|Texas Instruments Incorporated
| IBIS Model of : TMUX6213
| 48V 4x1:1 Analog Switch Array
| This file contains package information for the following:
|  TSSOP 16-pin (PW) package as [Component] TMUX6213_PW
|  QFN 16-pin (RUM) package as [Component] TMUX6213_RUM
| This device can be powered at the following Vccs:
| Single Rail Supply Configurations:
|  5.0 volt VDD, 0V VSS
|  12.0 volt VDD, 0V VSS
|  36.0 volt VDD, 0V VSS
| Dual Rail Supply Configurations:
|  5.0 volt VDD, -5V VSS
|  15.0 volt VDD, -15V VSS
| Digital Voltage Range : 4.5-38.5
[IBIS Ver] 4.1
[File name] tmux6213.ibs
[File Rev] 1.0
[Date] 12/30/2020
[Source]
| Texas Instruments Incorporated.
| 12500 TI Blvd
| Dallas, TX -75243
[Notes] Revision History:
| Rev 1.0: 12/30/2020
| - Initial version of the model
| - Model generated from simulations in TISPICE/SPECTRE
| - C_comp although listed in numerical order of value are
| obtained from varying PVT conditions. For PVT conditions for
| each specific value refer the buffer description under
| respective [Model]. IBIS model user is responsible for using
| appropriate C_comp to simulate for Signal Integrity.
| - Warnings regarding combined Non-monotonicity of various models have been
| reviewed and considered minor and can be ignored.
|**** Modify the following if you use [Model Selector]***********
| - Model names with a trailing voltage extension contain the model for
| operation at that voltage range.
[Disclaimer]
| This model is designed as an aid for customers of Texas Instruments.
| TI and its licensors and suppliers make no warranties, either expressed
| or implied, with respect to this model, including the warranties of
| merchantability or fitness for a particular purpose. The model is
| provided solely on an "as is" basis. The entire risk as to its quality
| and performance is with the customer.
| This model is subject to change without notice. Texas Instruments
| Incorporated is not responsible for updating this model.
[Copyright]
(C) Copyright 2020 Texas Instruments Incorporated. All rights reserved.
| Component TMUX6213_DGK 8-pin SOT (per package)
[Component] TMUX6213_PW
[Manufacturer]  Texas Instruments Incorporated
[Package] |TSSOP (PW) 16-pin
| variable typ min max
R_pkg 0.05 0.04 0.06
L_pkg 1.0nH 0.8nH 1.2nH
C_pkg 0.2pF 0.16pF 0.24pF
| pin number (pin name) mapping to model name
[Pin] signal_name   model_name   R_pin L_pin C_pin
1   IN1 		INPUT_PD   NA   NA   NA
2   D1   TMUX6213_DX   NA   NA   NA
3   S1   TMUX6213_SX   NA   NA   NA
4   VSS   POWER   NA   NA   NA
5   GND 		GND   NA   NA   NA
6   S4   TMUX6213_SX   NA   NA   NA
7   D4   TMUX6213_DX   NA   NA   NA
8   IN4 		INPUT_PD   NA   NA   NA
9   IN3 		INPUT_PD   NA   NA   NA
10   D3   TMUX6213_DX   NA   NA   NA
11   S3   TMUX6213_SX   NA   NA   NA
12   NC   NC   NA   NA   NA
13   VDD 		POWER   NA   NA   NA
14   S2   TMUX6213_SX   NA   NA   NA
15   D2   TMUX6213_DX   NA   NA   NA
16   IN2 		INPUT_PD   NA   NA   NA
[Series Switch Groups]
| Function Group States
On  1 /   | S1->D1 IN HIGH
Off  /   | EN LOW
[Series Pin Mapping]   pin_2   model_name   function_table_group
| PW Package
|2   3   TMUX6213_SX_SINGLE_5V_S   1
|3   2   TMUX6213_DX_SINGLE_5V_S   1
|15   14   TMUX6213_SX_SINGLE_5V_S   1
|14   15   TMUX6213_DX_SINGLE_5V_S   1
|7   6   TMUX6213_SX_SINGLE_5V_S   1
|6   7   TMUX6213_DX_SINGLE_5V_S   1
|10   11   TMUX6213_SX_SINGLE_5V_S   1
|11   10   TMUX6213_DX_SINGLE_5V_S   1
|2   3   TMUX6213_SX_SINGLE_12V_S   1
|3   2   TMUX6213_DX_SINGLE_12V_S   1
|15   14   TMUX6213_SX_SINGLE_12V_S   1
|14   15   TMUX6213_DX_SINGLE_12V_S   1
|7   6   TMUX6213_SX_SINGLE_12V_S   1
|6   7   TMUX6213_DX_SINGLE_12V_S   1
|10   11   TMUX6213_SX_SINGLE_12V_S   1
|11   10   TMUX6213_DX_SINGLE_12V_S   1
|2   3   TMUX6213_SX_SINGLE_36V_S   1
|3   2   TMUX6213_DX_SINGLE_36V_S   1
|15   14   TMUX6213_SX_SINGLE_36V_S   1
|14   15   TMUX6213_DX_SINGLE_36V_S   1
|7   6   TMUX6213_SX_SINGLE_36V_S   1
|6   7   TMUX6213_DX_SINGLE_36V_S   1
|10   11   TMUX6213_SX_SINGLE_36V_S   1
|11   10   TMUX6213_DX_SINGLE_36V_S   1
2   3   TMUX6213_SX_DUAL_PM5_S   1
3   2   TMUX6213_DX_DUAL_PM5_S   1
15   14   TMUX6213_SX_DUAL_PM5_S   1
14   15   TMUX6213_DX_DUAL_PM5_S   1
7   6   TMUX6213_SX_DUAL_PM5_S   1
6   7   TMUX6213_DX_DUAL_PM5_S   1
10   11   TMUX6213_SX_DUAL_PM5_S   1
11   10   TMUX6213_DX_DUAL_PM5_S   1
|2   3   TMUX6213_SX_DUAL_PM15_S   1
|3   2   TMUX6213_DX_DUAL_PM15_S   1
|15   14   TMUX6213_SX_DUAL_PM15_S   1
|14   15   TMUX6213_DX_DUAL_PM15_S   1
|7   6   TMUX6213_SX_DUAL_PM15_S   1
|6   7   TMUX6213_DX_DUAL_PM15_S   1
|10   11   TMUX6213_SX_DUAL_PM15_S   1
|11   10   TMUX6213_DX_DUAL_PM15_S   1
| Component TMUX6213_RUM 16-pin QFN (per package)
[Component] TMUX6213_RUM
[Manufacturer]  Texas Instruments Incorporated
[Package] |QFN (RUM) 16-pin
| variable typ 		min 		max
R_pkg 	0.05 		0.04 		0.06
L_pkg 	1.0nH 	0.8nH 	1.2nH
C_pkg 	0.2pF 	0.16pF 	0.24pF
| pin number (pin name) mapping to model name
[Pin] signal_name   model_name   R_pin L_pin C_pin
1   S1   TMUX6213_SX   NA   NA   NA
2   VSS   POWER   NA   NA   NA
3   GND 		GND   NA   NA   NA
4   S4   TMUX6213_SX   NA   NA   NA
5   D4   TMUX6213_DX   NA   NA   NA
6   IN4 		INPUT_PD   NA   NA   NA
7   IN3 		INPUT_PD   NA   NA   NA
8   D3   TMUX6213_DX   NA   NA   NA
9   S3   TMUX6213_SX   NA   NA   NA
10   NC   NC   NA   NA   NA
11   VDD 		POWER   NA   NA   NA
12   S2   TMUX6213_SX   NA   NA   NA
13   D2   TMUX6213_DX   NA   NA   NA
14   IN2 		INPUT_PD   NA   NA   NA
15   IN1 		INPUT_PD   NA   NA   NA
16   D1   TMUX6213_DX   NA   NA   NA
[Series Switch Groups]
| Function Group States
|On  1 /   | S1->D1 IN HIGH
|Off  /   | EN LOW
[Series Pin Mapping]   pin_2   model_name   function_table_group
| RUM Package
|16   1   TMUX6213_SX_SINGLE_5V_S   1
|1   16   TMUX6213_DX_SINGLE_5V_S   1
|13   12   TMUX6213_SX_SINGLE_5V_S   1
|12   13   TMUX6213_DX_SINGLE_5V_S   1
|8   8   TMUX6213_SX_SINGLE_5V_S   1
|9   9   TMUX6213_DX_SINGLE_5V_S   1
|5   4   TMUX6213_SX_SINGLE_5V_S   1
|4   5   TMUX6213_DX_SINGLE_5V_S   1
|16   1   TMUX6213_SX_SINGLE_12V_S   1
|1   16   TMUX6213_DX_SINGLE_12V_S   1
|13   12   TMUX6213_SX_SINGLE_12V_S   1
|12   13   TMUX6213_DX_SINGLE_12V_S   1
|8   8   TMUX6213_SX_SINGLE_12V_S   1
|9   9   TMUX6213_DX_SINGLE_12V_S   1
|5   4   TMUX6213_SX_SINGLE_12V_S   1
|4   5   TMUX6213_DX_SINGLE_12V_S   1
|16   1   TMUX6213_SX_SINGLE_36V_S   1
|1   16   TMUX6213_DX_SINGLE_36V_S   1
|13   12   TMUX6213_SX_SINGLE_36V_S   1
|12   13   TMUX6213_DX_SINGLE_36V_S   1
|8   8   TMUX6213_SX_SINGLE_36V_S   1
|9   9   TMUX6213_DX_SINGLE_36V_S   1
|5   4   TMUX6213_SX_SINGLE_36V_S   1
|4   5   TMUX6213_DX_SINGLE_36V_S   1
|16   1   TMUX6213_SX_DUAL_PM5_S   1
|1   16   TMUX6213_DX_DUAL_PM5_S   1
|13   12   TMUX6213_SX_DUAL_PM5_S   1
|12   13   TMUX6213_DX_DUAL_PM5_S   1
|8   8   TMUX6213_SX_DUAL_PM5_S   1
|9   9   TMUX6213_DX_DUAL_PM5_S   1
|5   4   TMUX6213_SX_DUAL_PM5_S   1
|4   5   TMUX6213_DX_DUAL_PM5_S   1
|16   1   TMUX6213_SX_DUAL_PM15_S   1
|1   16   TMUX6213_DX_DUAL_PM15_S   1
|13   12   TMUX6213_SX_DUAL_PM15_S   1
|12   13   TMUX6213_DX_DUAL_PM15_S   1
|8   8   TMUX6213_SX_DUAL_PM15_S   1
|9   9   TMUX6213_DX_DUAL_PM15_S   1
|5   4   TMUX6213_SX_DUAL_PM15_S   1
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[Model Selector] INPUT_PU
INBUF_PU_5V   INPUT_PU   buffer at 5V operation.
INBUF_PU_12V   INPUT_PU   buffer at 12V operation.
INBUF_PU_15V   INPUT_PU   buffer at 15V operation.
INBUF_PU_20V   INPUT_PU   buffer at 20V operation.
INBUF_PU_36V   INPUT_PU   buffer at 36V operation.
[Model Selector] INPUT_PD
INBUF_PD_5V   INPUT_PD   buffer at 5V operation.
INBUF_PD_12V   INPUT_PD   buffer at 12V operation.
INBUF_PD_15V   INPUT_PD   buffer at 15V operation.
INBUF_PD_20V   INPUT_PD   buffer at 20V operation.
INBUF_PD_36V   INPUT_PD   buffer at 36V operation.
[Model Selector] TMUX6213_SX
TMUX6213_SX_SINGLE_5V  switch termination at +5V operation.
TMUX6213_SX_SINGLE_12V  switch termination at +12V operation.
TMUX6213_SX_SINGLE_36V  switch termination at +36V operation.
TMUX6213_SX_DUAL_PM5  switch termination at +/-5V operation.
TMUX6213_SX_DUAL_PM15  switch termination at +/-15V operation.
[Model Selector] TMUX6213_SX_S
TMUX6213_SX_SINGLE_5V_S  switch at +5V operation.
TMUX6213_SX_SINGLE_12V_S  switch at +12V operation.
TMUX6213_SX_SINGLE_36V_S  switch at +36V operation.
TMUX6213_SX_DUAL_PM5_S  switch at +/-5V operation.
TMUX6213_SX_DUAL_PM15_S  switch at +/-15V operation.
[Model Selector] TMUX6213_DX
TMUX6213_DX_SINGLE_5V  termination switch at +5V operation.
TMUX6213_DX_SINGLE_12V  termination switch at +12V operation.
TMUX6213_DX_SINGLE_36V  termination switch at +36V operation.
TMUX6213_DX_DUAL_PM5	termination switch at +/-15V operation.
TMUX6213_DX_DUAL_PM15  termination switch at +/-15V operation.
[Model Selector] TMUX6213_DX_S
TMUX6213_DX_SINGLE_5V_S  switch at +5V operation.
TMUX6213_DX_SINGLE_12V_S  switch at +12V operation.
TMUX6213_DX_SINGLE_36V_S  switch at +36V operation.
TMUX6213_DX_DUAL_PM5_S  switch at +/-5V operation.
TMUX6213_DX_DUAL_PM15_S  switch at +/-15V operation.
| Model12
[Model]   TMUX6213_SX_SINGLE_5V_S
Model_type  Series_switch
| variable   typ   min   max
C_comp   0   0   0
[Temperature Range]   25   125   -40
| Ambient temperature   25   125   -40
[Voltage range]   5   4.5   5.5
[On]
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[Off]
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[Model]   TMUX6213_DX_SINGLE_5V_S
Model_type  Series_switch
| variable   typ   min   max
C_comp   0   0   0
[Temperature Range]   25   125   -40
| Ambient temperature   25   125   -40
[Voltage range]   5   5   5
[On]
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[Off]
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[Model]   TMUX6213_SX_SINGLE_12V_S
Model_type  Series_switch
| variable   typ   min   max
C_comp   0   0   0
[Temperature Range]   25   125   -40
| Ambient temperature   25   125   -40
[Voltage range]   12   12   12
[On]
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[Off]
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[Model]   TMUX6213_DX_SINGLE_12V_S
Model_type  Series_switch
| variable   typ   min   max
C_comp   0   0   0
[Temperature Range]   25   125   -40
| Ambient temperature   25   125   -40
[Voltage range]   12   12   12
[On]
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[Off]
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[Model]   TMUX6213_SX_SINGLE_36V_S
Model_type  Series_switch
| variable   typ   min   max
C_comp   0   0   0
[Temperature Range]   25   125   -40
| Ambient temperature   25   125   -40
[Voltage range]   36   36   36
[On]
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[Off]
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[Model]   TMUX6213_DX_SINGLE_36V_S
Model_type  Series_switch
| variable   typ   min   max
C_comp   0   0   0
[Temperature Range]   25   125   -40
| Ambient temperature   25   125   -40
[Voltage range]   36   36   36
[On]
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[Off]
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[Model]   TMUX6213_SX_DUAL_PM5_S
Model_type  Series_switch
| variable   typ   min   max
C_comp   0   0   0
[Temperature Range]   25   125   -40
| Ambient temperature   25   125   -40
[Voltage range]   0   -5   5
[On]
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[Off]
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[Model]   TMUX6213_DX_DUAL_PM5_S
Model_type  Series_switch
| variable   typ   min   max
C_comp   0   0   0
[Temperature Range]   25   125   -40
| Ambient temperature   25   125   -40
[Voltage range]   0   -5   5
[On]
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[Off]
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[Model]   TMUX6213_SX_DUAL_PM15_S
Model_type  Series_switch
| variable   typ   min   max
C_comp   0   0   0
[Temperature Range]   25   125   -40
| Ambient temperature   25   125   -40
[Voltage range]   0   -15   15
[On]
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[Off]
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[Model]   TMUX6213_DX_DUAL_PM15_S
Model_type  Series_switch
| variable   typ   min   max
C_comp   0   0   0
[Temperature Range]   25   125   -40
| Ambient temperature   25   125   -40
[Voltage range]   0   -15   15
[On]
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[Off]
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| Models and submodels in the file (30): INBUF_PD_5V (Input), INBUF_PD_12V (Input), INBUF_PD_15V (Input), INBUF_PD_20V (Input), INBUF_PD_36V (Input), INBUF_PU_5V (Input), INBUF_PU_12V (Input), INBUF_PU_15V (Input), INBUF_PU_20V (Input), INBUF_PU_36V (Input), TMUX6213_SX_SINGLE_5V_S (Series_switch), TMUX6213_SX_SINGLE_5V (Terminator), TMUX6213_DX_SINGLE_5V_S (Series_switch), TMUX6213_DX_SINGLE_5V (Terminator), TMUX6213_SX_SINGLE_12V_S (Series_switch), TMUX6213_SX_SINGLE_12V (Terminator), TMUX6213_DX_SINGLE_12V_S (Series_switch), TMUX6213_DX_SINGLE_12V (Terminator), TMUX6213_SX_SINGLE_36V_S (Series_switch), TMUX6213_SX_SINGLE_36V (Terminator), TMUX6213_DX_SINGLE_36V_S (Series_switch), TMUX6213_DX_SINGLE_36V (Terminator), TMUX6213_SX_DUAL_PM5_S (Series_switch), TMUX6213_SX_DUAL_PM5 (Terminator), TMUX6213_DX_DUAL_PM5_S (Series_switch), TMUX6213_DX_DUAL_PM5 (Terminator), TMUX6213_SX_DUAL_PM15_S (Series_switch), TMUX6213_SX_DUAL_PM15 (Terminator), TMUX6213_DX_DUAL_PM15_S (Series_switch), TMUX6213_DX_DUAL_PM15 (Terminator)
